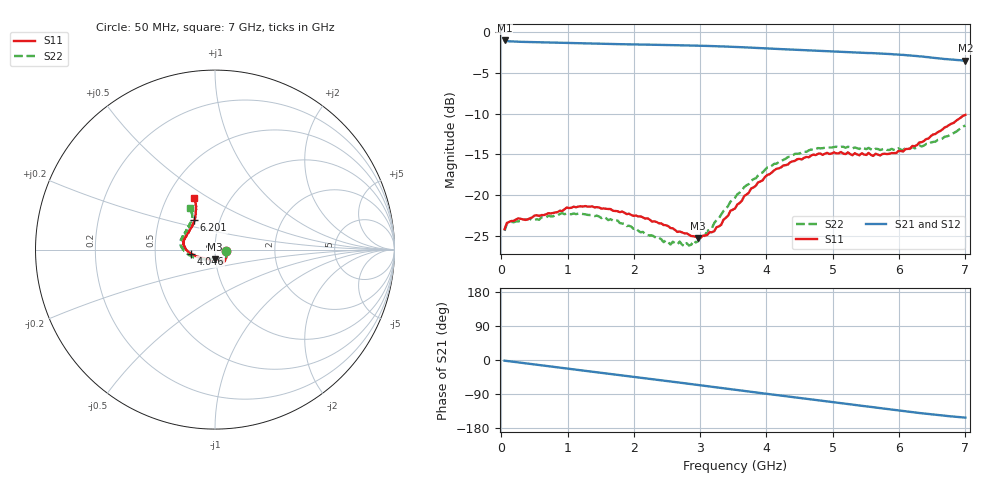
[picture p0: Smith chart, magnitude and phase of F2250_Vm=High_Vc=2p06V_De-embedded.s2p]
! Integrated Device Technology
! Corporate Headquarters
! 6024 Silver Creek Valley Road
! San Jose, CA 95138  USA
! Phone:  1-408-284-8200
! Toll Free:  1-800-223-1366
! Webpage:  http://www.idt.com/
! Timing and RF Division
! 515 Groton Road, Suite 102
! Westford, MA 01886-6024
! Device:  F2250
! Description: Voltage Variable RF Attenuator
! Frequency:  50.0 -  6000.00 MHz
! Package:  3x3 mm Thin QFN Plastic Package: 16 pin
! Ports:  2 RF, 3 DC
!  Pin  1  = GND
!  Pin  2  = NC
!  Pin  3  = RF1  = Port 1
!  Pin  4  = NC
!  Pin  5  = GND
!  Pin  6  = GND
!  Pin  7  = GND
!  Pin  8  = GND
!  Pin  9  = NC
!  Pin 10  = RF2  = Port 2
!  Pin 11  = NC
!  Pin 12  = GND
!  Pin 13  = GND
!  Pin 14  = VCNTRL
!  Pin 15  = VDD
!  Pin 16  = VMODE
! Vcntrl:  2.060 Volts
! Vmode:  +3.300 Volts
! Vdd:  +3.30  Volts
! Current:  1.321 mA
! Data:  The device was measured on a the F2250 evaluation board which has
!  individual transmission lines to the RF pins.  Data was collected
!  using a calibrated network analyzer.  The evaluation board was
!  de-embedded using a TRL calibration technique.
!  The reference plane is the edge of the package pin.
! Misc:  SN 10
!  Action Tracker AT0258
! Date Measured:  2014-11-26
! Date:  2015-10-15  MJV
! Note:
!  Integrated Device Technology supplies this data as a sample of measured
!  data at the package pin for this product.  Your particular data for this
!  product may vary.
!  Data was taken at 25 degrees C.
!  Integrated Device Technology reserves the right to change this data at anytime.
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# GHz S dB R 50
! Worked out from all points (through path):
!   201 points, 50 MHz to 7 GHz, reference 50 ohm
!   highest |S21| = -0.98 dB at 50 MHz (marker M1); lowest = -3.5 dB at 7 GHz (marker M2)
!   group delay of S21, straight-line fit = 61.1 ps
!   lowest |S11| = -25.3 dB at 2.969 GHz (marker M3), VSWR 1.12, Z = 49.8 - j5.45 ohm
!   |S11| at or under -10 dB: start of sweep to end of sweep
!   |S22| runs from -26.3 to -11.4 dB; largest |S21 - S12| = 0.0019
!   S11 on the Smith chart (normalised r, x): 50 MHz: 1.13, -0.02; 4.046 GHz: 0.77, -0.04; 6.201 GHz: 0.75, +0.26; 7 GHz: 0.68, +0.43
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0.05  -24.19 -9.1  -0.98 -1.8  -0.98 -1.8  -24.39 -9.7
0.08475  -23.41 -8.3  -1.06 -2.5  -1.06 -2.5  -23.50 -8.7
0.1195  -23.29 -8.9  -1.09 -3.3  -1.09 -3.2  -23.31 -8.1
0.91875  -21.95 -45.5  -1.28 -21.0  -1.28 -21.1  -22.22 -48.3
1.2315  -21.40 -53.3  -1.34 -27.9  -1.34 -27.9  -22.33 -58.7
1.75275  -21.98 -60.1  -1.44 -39.1  -1.44 -39.1  -23.12 -66.3
2.37825  -23.47 -60.5  -1.53 -52.7  -1.53 -52.8  -25.24 -69.1
2.552  -24.05 -64.9  -1.55 -56.6  -1.55 -56.6  -26.08 -75.6
2.691  -24.48 -71.9  -1.57 -59.7  -1.57 -59.7  -25.71 -82.7
2.7605  -24.70 -73.8  -1.59 -61.3  -1.59 -61.3  -26.28 -87.0
2.969  -25.25 -89.3  -1.63 -65.9  -1.63 -66.0  -25.67 -104.4
3.21225  -24.43 -118.2  -1.68 -71.4  -1.68 -71.5  -23.42 -127.8
3.525  -21.64 -145.6  -1.78 -78.5  -1.78 -78.5  -20.32 -146.5
3.76825  -19.19 -159.6  -1.87 -84.0  -1.87 -84.0  -18.24 -157.9
4.04625  -17.43 -170.0  -1.98 -90.2  -1.98 -90.2  -16.59 -168.5
4.4285  -15.79 179.3  -2.13 -98.6  -2.13 -98.6  -14.93 179.9
4.7065  -15.02 172.0  -2.23 -104.8  -2.23 -104.8  -14.44 173.9
5.054  -14.87 163.8  -2.36 -112.4  -2.35 -112.5  -14.05 166.7
5.85325  -14.92 137.5  -2.65 -129.9  -2.65 -130.0  -14.45 147.8
6.20075  -13.96 125.5  -2.86 -137.7  -2.86 -137.7  -14.06 138.6
6.54825  -12.48 117.2  -3.13 -144.7  -3.13 -144.8  -13.42 127.2
7  -10.14 112.0  -3.46 -152.0  -3.47 -152.1  -11.44 120.9
